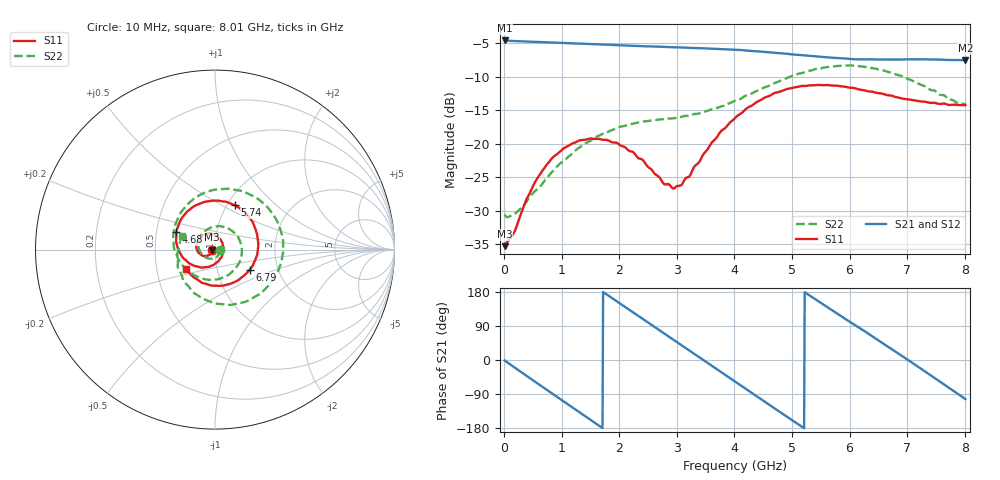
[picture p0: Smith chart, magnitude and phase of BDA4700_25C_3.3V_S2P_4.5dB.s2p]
!Agilent Technologies,E5071B,MY42404982,A.09.10
!Date: Mon Oct 20 18:04:52 2025
!Data & Calibration Information:
!Freq	S11:SOLT2(ON)	S21:SOLT2(ON)	S12:SOLT2(ON)	S22:SOLT2(ON)
# Hz S RI R 50
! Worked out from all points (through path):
!   801 points, 10 MHz to 8.01 GHz, reference 50 ohm
!   highest |S21| = -4.62 dB at 10 MHz (marker M1); lowest = -7.6 dB at 8.01 GHz (marker M2)
!   group delay of S21, straight-line fit = 284 ps
!   lowest |S11| = -35.3 dB at 10 MHz (marker M3), VSWR 1.03, Z = 48.3 - j0.12 ohm
!   |S11| at or under -10 dB: start of sweep to end of sweep
!   |S22| runs from -31.0 to -8.3 dB; largest |S21 - S12| = 0.0067
!   S11 on the Smith chart (normalised r, x): 10 MHz: 0.97, -0.00; 4.68 GHz: 0.63, +0.13; 5.74 GHz: 1.09, +0.58; 6.79 GHz: 1.43, -0.34; 8.01 GHz: 0.71, -0.16
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1e7  -0.0171 -0.00124  0.5873 -0.0124  0.5872 -0.013  0.0295 -0.0025
3.3e8  -0.0242 -0.0225  0.472 -0.3343  0.4717 -0.3346  0.0209 -0.0268
7.2e8  -0.057 -0.0361  0.1345 -0.5541  0.1347 -0.5539  -0.0181 -0.0509
1.02e9  -0.0883 -0.0206  -0.1715 -0.537  -0.1716 -0.537  -0.0638 -0.036
1.35e9  -0.1044 0.019  -0.4391 -0.3414  -0.4394 -0.3417  -0.0924 0.0256
1.93e9  -0.0564 0.0847  -0.502 0.2064  -0.5022 0.2062  0.00219 0.1286
2.32e9  0.00127 0.0785  -0.2471 0.4736  -0.2471 0.474  0.1099 0.0917
2.68e9  0.0403 0.0401  0.087 0.5206  0.0861 0.5201  0.1498 -0.0175
2.96e9  0.0458 -0.0067  0.3231 0.4102  0.3229 0.4096  0.1149 -0.1037
3.37e9  0.0116 -0.0701  0.5074 0.0854  0.5082 0.0858  -0.00641 -0.1666
4.01e9  -0.1302 -0.0837  0.2756 -0.4177  0.2762 -0.4171  -0.1983 -0.0639
4.34e9  -0.1965 -0.015  -0.0058 -0.4885  -0.00586 -0.4899  -0.2327 0.0628
4.68e9  -0.216 0.0966  -0.2785 -0.3855  -0.2775 -0.3868  -0.1907 0.2059
5.02e9  -0.1601 0.2064  -0.4354 -0.1536  -0.4366 -0.1544  -0.061 0.3154
5.35e9  -0.0461 0.2679  -0.4355 0.11  -0.4361 0.1074  0.1181 0.3315
5.74e9  0.1116 0.2464  -0.2616 0.3483  -0.2608 0.348  0.3107 0.2138
6.19e9  0.2272 0.1089  0.0538 0.4202  0.0594 0.4209  0.373 -0.0493
6.68e9  0.2152 -0.0781  0.3519 0.2347  0.3528 0.2339  0.2031 -0.274
6.79e9  0.1923 -0.1126  0.39 0.1637  0.391 0.1611  0.1465 -0.2957
7.31e9  0.0347 -0.202  0.3663 -0.2149  0.3663 -0.2156  -0.1201 -0.2393
7.66e9  -0.0784 -0.1815  0.167 -0.386  0.1664 -0.3867  -0.2076 -0.0889
8.01e9  -0.1601 -0.1094  -0.0957 -0.4066  -0.0945 -0.4069  -0.1813 0.0754
